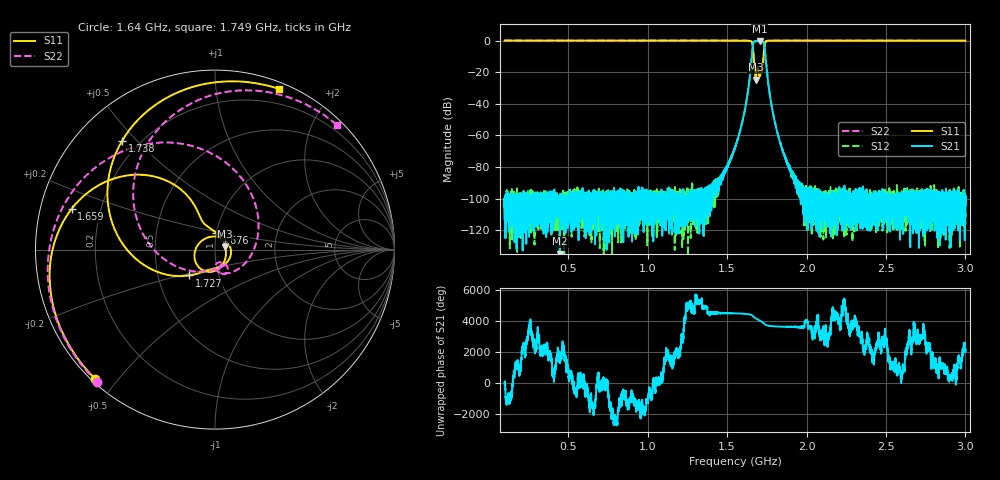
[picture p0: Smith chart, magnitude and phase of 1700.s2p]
# Hz S DB R 50
! Planar, S50180, 20087770, 20.1.2/1
! Date: 23.06.2021 14:46:07
! Data: Format (Calibration Info)
! Freq	S11:dB/Ang(F2)	S21:dB/Ang(F2)	S12:dB/Ang(F2)	S22:dB/Ang(F2)
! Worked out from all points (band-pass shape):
!   8991 points, 100 MHz to 3 GHz, reference 50 ohm
!   highest |S21| = -0.36 dB at 1.705 GHz (marker M1); lowest = -134.6 dB at 448.4 MHz (marker M2)
!   |S21| within 3 dB of the highest: 1.662 GHz to 1.735 GHz (72.68 MHz wide, 4.28 % of centre)
!   lowest |S11| = -24.7 dB at 1.68 GHz (marker M3), VSWR 1.12, Z = 55.9 + j1.93 ohm
!   |S11| at or under -10 dB: 1.667 GHz to 1.729 GHz (62.5 MHz wide, 3.68 % of centre)
!   |S22| runs from -22.6 to 0.0 dB; largest |S21 - S12| = 0.0025
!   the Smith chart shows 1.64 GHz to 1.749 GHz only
!   S11 on the Smith chart (normalised r, x): 1.64 GHz: 0.01, -0.44; 1.659 GHz: 0.09, +0.14; 1.676 GHz: 0.99, +0.19; 1.727 GHz: 0.72, -0.22; 1.738 GHz: 0.14, +0.45; 1.749 GHz: 0.06, +1.47
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1e8  0.02 154.0  -104.92 95.7  -105.07 113.0  0.01 150.1
4.483871e8  -0.02 77.2  -134.62 107.3  -121.02 162.9  0.01 68.4
5.835484e8  -0.01 55.2  -112.34 46.5  -105.92 -141.0  0.01 45.9
1.066774e9  0.00 -5.7  -102.52 173.1  -101.98 27.2  0.04 -11.6
1.488387e9  -0.01 -57.7  -82.53 -146.4  -82.50 -160.8  0.02 -58.8
1.55e9  -0.03 -71.7  -67.62 -161.0  -67.76 -162.5  0.00 -71.5
1.603226e9  -0.05 -94.2  -48.27 175.6  -48.26 175.3  -0.04 -92.2
1.640323e9  -0.16 -132.9  -25.50 135.4  -25.51 135.3  -0.11 -131.7
1.65871e9  -1.62 164.1  -6.65 61.9  -6.67 61.8  -1.78 147.0
1.676452e9  -20.46 86.9  -0.44 -94.1  -0.44 -94.1  -19.58 -88.7
1.680323e9  -24.68 17.1  -0.39 -119.8  -0.40 -119.9  -22.59 -74.2
1.691935e9  -17.47 -128.6  -0.42 170.2  -0.43 170.1  -16.67 -67.9
1.704516e9  -22.75 83.1  -0.36 98.0  -0.37 98.0  -20.95 -65.9
1.715806e9  -20.25 -52.8  -0.40 30.3  -0.41 30.2  -19.78 -64.4
1.726774e9  -13.82 -135.0  -0.66 -47.3  -0.67 -47.4  -14.16 -144.7
1.737742e9  -1.98 130.6  -5.90 -149.2  -5.91 -149.3  -1.93 104.2
1.74871e9  -0.32 68.4  -17.43 149.5  -17.45 149.4  -0.26 45.5
1.779032e9  -0.06 9.9  -40.43 93.8  -40.43 93.7  -0.06 -5.1
1.877419e9  -0.03 -36.4  -76.45 52.3  -77.36 47.3  0.02 -43.4
2.033548e9  -0.04 -60.9  -98.69 -16.7  -102.19 107.0  -0.01 -64.7
2.516774e9  -0.07 -103.3  -110.26 160.8  -102.44 -94.2  -0.05 -102.9
3e9  -0.11 -138.9  -104.21 -24.4  -112.13 176.6  -0.09 -136.0
